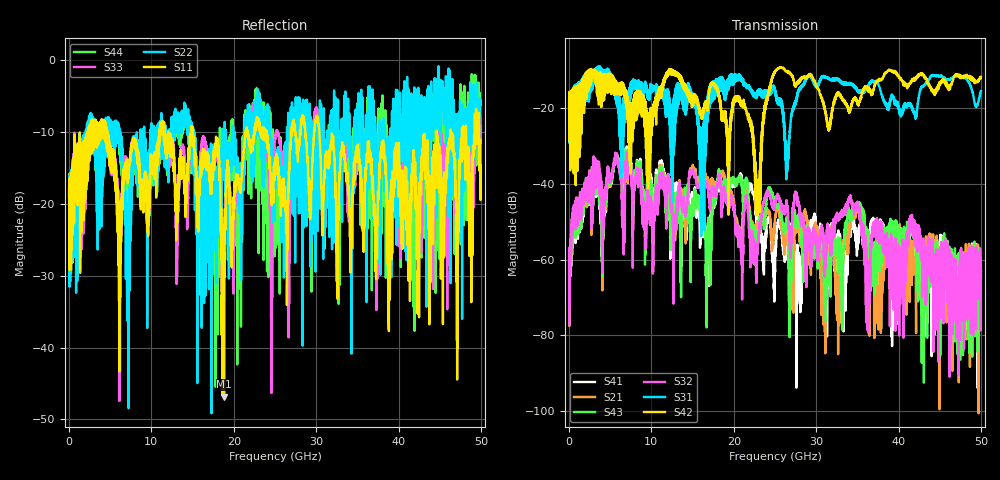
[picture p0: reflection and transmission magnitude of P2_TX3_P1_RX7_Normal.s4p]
!Keysight Technologies,N5225B,MY57041031,A.13.20.10
!Date: Friday, May 31, 2019 11:25:01
!Correction: S11(Full 4 Port(1,2,3,4))
!S12(Full 4 Port(1,2,3,4))
!S13(Full 4 Port(1,2,3,4))
!S14(Full 4 Port(1,2,3,4))
!S21(Full 4 Port(1,2,3,4))
!S22(Full 4 Port(1,2,3,4))
!S23(Full 4 Port(1,2,3,4))
!S24(Full 4 Port(1,2,3,4))
!S31(Full 4 Port(1,2,3,4))
!S32(Full 4 Port(1,2,3,4))
!S33(Full 4 Port(1,2,3,4))
!S34(Full 4 Port(1,2,3,4))
!S41(Full 4 Port(1,2,3,4))
!S42(Full 4 Port(1,2,3,4))
!S43(Full 4 Port(1,2,3,4))
!S44(Full 4 Port(1,2,3,4))
!S4P File: Measurements: <S11,S12,S13,S14>,
!<S21,S22,S23,S24>,
!<S31,S32,S33,S34>,
!<S41,S42,S43,S44>:
# Hz S  dB  R 50.0
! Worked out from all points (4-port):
!   5000 points, 10 MHz to 50 GHz, reference 50 ohm
!   strongest paths, dB at 10 MHz, 12.51 GHz, 25.01 GHz, 37.51 GHz, 50 GHz:
!     S42: -19.6, -9.9, -10.6, -12.6, -11.8
!     S31: -19.6, -43.4, -16.0, -13.6, -15.6
!     S32: -56.9, -46.0, -44.9, -50.6, -65.0
!     S43: -57.3, -49.8, -45.6, -57.2, -61.4
!     S21: -61.1, -47.8, -48.7, -69.3, -63.2
!     S41: -64.2, -47.6, -63.3, -51.7, -64.6
!   lowest |S11| = -46.8 dB at 18.82 GHz (marker M1), VSWR 1.01, Z = 49.6 + j0.0866 ohm
!   |S11| at or under -10 dB: 4.63 GHz to 10.95 GHz (6.318 GHz wide, 81.1 % of centre); 15.04 GHz to 21.46 GHz (6.426 GHz wide, 35.2 % of centre); 30.38 GHz to 44.61 GHz (14.22 GHz wide, 37.9 % of centre)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
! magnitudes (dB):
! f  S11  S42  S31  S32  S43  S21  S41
! 10 MHz  -19.6  -19.6  -19.6  -56.9  -57.3  -61.1  -64.2
! 5.72 GHz  -19.1  -16.2  -16.9  -32.0  -32.2  -31.9  -32.2
! 16.86 GHz  -14.5  -19.1  -21.7  -40.6  -53.4  -38.5  -56.4
! 18.82 GHz  -46.8  -23.0  -13.3  -41.1  -40.3  -37.9  -38.9
! 22.93 GHz  -8.6  -40.7  -15.7  -55.9  -54.4  -51.4  -49.0
! 25.48 GHz  -16.1  -9.5  -17.5  -44.1  -45.8  -47.2  -50.1
! 50 GHz  -15.7  -11.8  -15.6  -65.0  -61.4  -63.2  -64.6
